FUNCTION "PALLET IMP.POST. SU USCI" : VOID
TITLE =
VERSION : 0.1
//KNOW_HOW_PROTECT

VAR_TEMP
  Error_block_move : INT ;
END_VAR
BEGIN
NETWORK
TITLE =

NETWORK
TITLE =Spostamento dati per pallet in transito tra ribaltat. e uscita
//- "Container Flag"
//- "Id TAG"
//- "FlagRibaltamento"
//- "Container_Id"
//- "Date LCB"
//- "Part Number"
//- "Quantity"
//- "Line Id"
//- "CIM"
//- "Colata Id"
//- "Material Of Test Flag"
//- "Lotto Id"
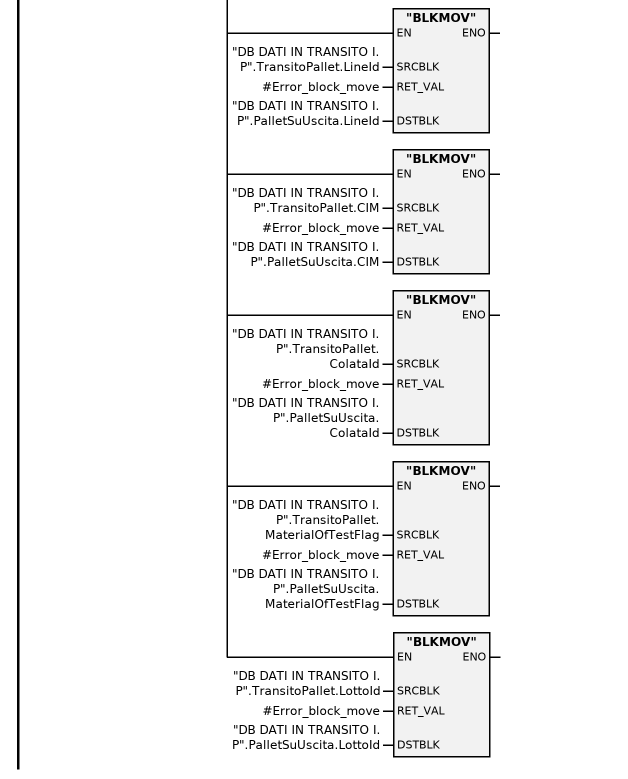
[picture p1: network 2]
      U     "M900.0";
      U     "DB SCAMBIO DATI PIANELLI".Pallet_I_P_su_uscita;
      =     L      2.0;
      U     L      2.0;
      SPBNB _001;
      CALL "BLKMOV" (
           SRCBLK                   := "DB DATI IN TRANSITO I. P".TransitoPallet.ContainerFlag,
           RET_VAL                  := #Error_block_move,
           DSTBLK                   := "DB DATI IN TRANSITO I. P".PalletSuUscita.ContainerFlag);
_001: NOP   0;
      U     L      2.0;
      SPBNB _002;
      CALL "BLKMOV" (
           SRCBLK                   := "DB DATI IN TRANSITO I. P".TransitoPallet.ID_TAG,
           RET_VAL                  := #Error_block_move,
           DSTBLK                   := "DB DATI IN TRANSITO I. P".PalletSuUscita.ID_TAG);
_002: NOP   0;
      U     L      2.0;
      SPBNB _003;
      CALL "BLKMOV" (
           SRCBLK                   := "DB DATI IN TRANSITO I. P".TransitoPallet.FlagRibaltamento,
           RET_VAL                  := #Error_block_move,
           DSTBLK                   := "DB DATI IN TRANSITO I. P".PalletSuUscita.FlagRibaltamento);
_003: NOP   0;
      U     L      2.0;
      SPBNB _004;
      CALL "BLKMOV" (
           SRCBLK                   := "DB DATI IN TRANSITO I. P".TransitoPallet.Container_Id,
           RET_VAL                  := #Error_block_move,
           DSTBLK                   := "DB DATI IN TRANSITO I. P".PalletSuUscita.Container_Id);
_004: NOP   0;
      U     L      2.0;
      SPBNB _005;
      CALL "BLKMOV" (
           SRCBLK                   := "DB DATI IN TRANSITO I. P".TransitoPallet.DateLCB,
           RET_VAL                  := #Error_block_move,
           DSTBLK                   := "DB DATI IN TRANSITO I. P".PalletSuUscita.DateLCB);
_005: NOP   0;
      U     L      2.0;
      SPBNB _006;
      CALL "BLKMOV" (
           SRCBLK                   := "DB DATI IN TRANSITO I. P".TransitoPallet.PartNumber,
           RET_VAL                  := #Error_block_move,
           DSTBLK                   := "DB DATI IN TRANSITO I. P".PalletSuUscita.PartNumber);
_006: NOP   0;
      U     L      2.0;
      SPBNB _007;
      CALL "BLKMOV" (
           SRCBLK                   := "DB DATI IN TRANSITO I. P".TransitoPallet.Quantity,
           RET_VAL                  := #Error_block_move,
           DSTBLK                   := "DB DATI IN TRANSITO I. P".PalletSuUscita.Quantity);
_007: NOP   0;
      U     L      2.0;
      SPBNB _008;
      CALL "BLKMOV" (
           SRCBLK                   := "DB DATI IN TRANSITO I. P".TransitoPallet.LineId,
           RET_VAL                  := #Error_block_move,
           DSTBLK                   := "DB DATI IN TRANSITO I. P".PalletSuUscita.LineId);
_008: NOP   0;
      U     L      2.0;
      SPBNB _009;
      CALL "BLKMOV" (
           SRCBLK                   := "DB DATI IN TRANSITO I. P".TransitoPallet.CIM,
           RET_VAL                  := #Error_block_move,
           DSTBLK                   := "DB DATI IN TRANSITO I. P".PalletSuUscita.CIM);
_009: NOP   0;
      U     L      2.0;
      SPBNB _00a;
      CALL "BLKMOV" (
           SRCBLK                   := "DB DATI IN TRANSITO I. P".TransitoPallet.ColataId,
           RET_VAL                  := #Error_block_move,
           DSTBLK                   := "DB DATI IN TRANSITO I. P".PalletSuUscita.ColataId);
_00a: NOP   0;
      U     L      2.0;
      SPBNB _00b;
      CALL "BLKMOV" (
           SRCBLK                   := "DB DATI IN TRANSITO I. P".TransitoPallet.MaterialOfTestFlag,
           RET_VAL                  := #Error_block_move,
           DSTBLK                   := "DB DATI IN TRANSITO I. P".PalletSuUscita.MaterialOfTestFlag);
_00b: NOP   0;
      U     L      2.0;
      SPBNB _00c;
      CALL "BLKMOV" (
           SRCBLK                   := "DB DATI IN TRANSITO I. P".TransitoPallet.LottoId,
           RET_VAL                  := #Error_block_move,
           DSTBLK                   := "DB DATI IN TRANSITO I. P".PalletSuUscita.LottoId);
_00c: NOP   0;
NETWORK
TITLE =Lettura Pallet su baia di scarico
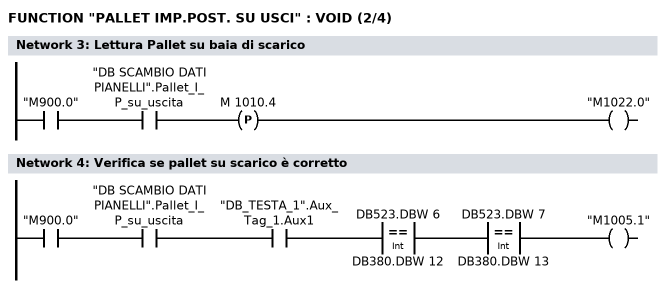
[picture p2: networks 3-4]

      U     "M900.0";
      U     "DB SCAMBIO DATI PIANELLI".Pallet_I_P_su_uscita;
      FP    M   1010.4;
      =     "M1022.0";
NETWORK
TITLE =Verifica se pallet su scarico è corretto

      U     "M900.0";
      U     "DB SCAMBIO DATI PIANELLI".Pallet_I_P_su_uscita;
      U     "DB_TESTA_1".Aux_Tag_1.Aux1;
      U(    ;
      L     DB523.DBW    6;
      L     DB380.DBW   12;
      ==I   ;
      )     ;
      U(    ;
      L     DB523.DBW    7;
      L     DB380.DBW   13;
      ==I   ;
      )     ;
      =     "M1005.1";
NETWORK
TITLE =Se pallet è corretto e ribaltato, aggiorno TAG
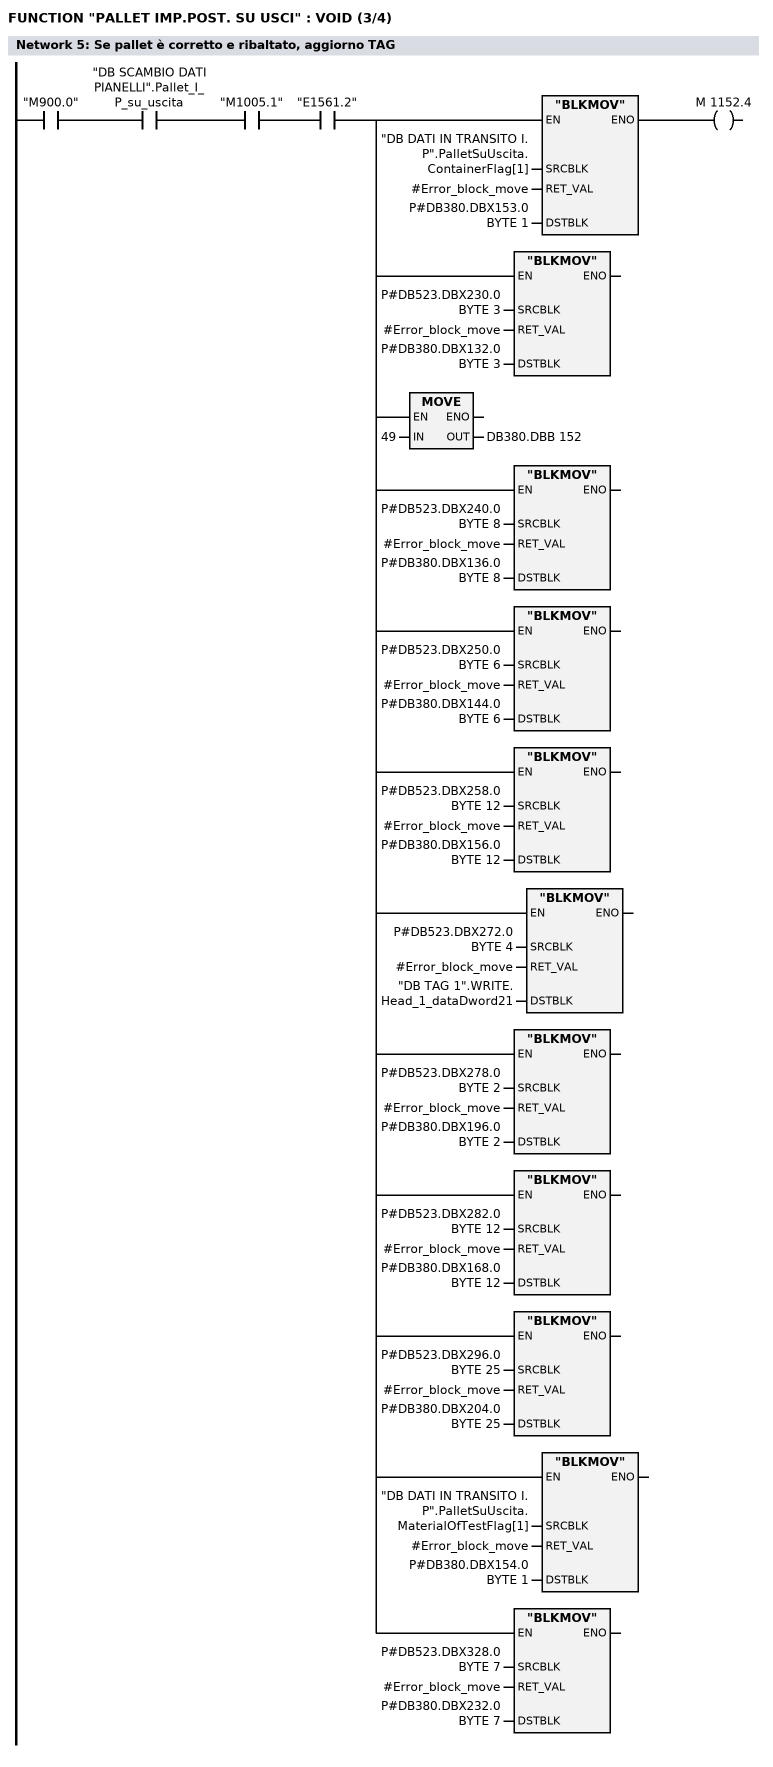
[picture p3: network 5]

      U     "M900.0";
      U     "DB SCAMBIO DATI PIANELLI".Pallet_I_P_su_uscita;
      U     "M1005.1";
      U     "E1561.2";
      =     L      2.0;
      U     L      2.0;
      SPBNB _00d;
      CALL "BLKMOV" (
           SRCBLK                   := "DB DATI IN TRANSITO I. P".PalletSuUscita.ContainerFlag[1],
           RET_VAL                  := #Error_block_move,
           DSTBLK                   := P#DB380.DBX153.0 BYTE 1);
_00d: U     BIE;
      =     M   1152.4;
      U     L      2.0;
      SPBNB _00e;
      CALL "BLKMOV" (
           SRCBLK                   := P#DB523.DBX230.0 BYTE 3,
           RET_VAL                  := #Error_block_move,
           DSTBLK                   := P#DB380.DBX132.0 BYTE 3);
_00e: NOP   0;
      U     L      2.0;
      SPBNB _00f;
      L     49;
      T     DB380.DBB  152;
_00f: NOP   0;
      U     L      2.0;
      SPBNB _010;
      CALL "BLKMOV" (
           SRCBLK                   := P#DB523.DBX240.0 BYTE 8,
           RET_VAL                  := #Error_block_move,
           DSTBLK                   := P#DB380.DBX136.0 BYTE 8);
_010: NOP   0;
      U     L      2.0;
      SPBNB _011;
      CALL "BLKMOV" (
           SRCBLK                   := P#DB523.DBX250.0 BYTE 6,
           RET_VAL                  := #Error_block_move,
           DSTBLK                   := P#DB380.DBX144.0 BYTE 6);
_011: NOP   0;
      U     L      2.0;
      SPBNB _012;
      CALL "BLKMOV" (
           SRCBLK                   := P#DB523.DBX258.0 BYTE 12,
           RET_VAL                  := #Error_block_move,
           DSTBLK                   := P#DB380.DBX156.0 BYTE 12);
_012: NOP   0;
      U     L      2.0;
      SPBNB _013;
      CALL "BLKMOV" (
           SRCBLK                   := P#DB523.DBX272.0 BYTE 4,
           RET_VAL                  := #Error_block_move,
           DSTBLK                   := "DB TAG 1".WRITE.Head_1_dataDword21);
_013: NOP   0;
      U     L      2.0;
      SPBNB _014;
      CALL "BLKMOV" (
           SRCBLK                   := P#DB523.DBX278.0 BYTE 2,
           RET_VAL                  := #Error_block_move,
           DSTBLK                   := P#DB380.DBX196.0 BYTE 2);
_014: NOP   0;
      U     L      2.0;
      SPBNB _015;
      CALL "BLKMOV" (
           SRCBLK                   := P#DB523.DBX282.0 BYTE 12,
           RET_VAL                  := #Error_block_move,
           DSTBLK                   := P#DB380.DBX168.0 BYTE 12);
_015: NOP   0;
      U     L      2.0;
      SPBNB _016;
      CALL "BLKMOV" (
           SRCBLK                   := P#DB523.DBX296.0 BYTE 25,
           RET_VAL                  := #Error_block_move,
           DSTBLK                   := P#DB380.DBX204.0 BYTE 25);
_016: NOP   0;
      U     L      2.0;
      SPBNB _017;
      CALL "BLKMOV" (
           SRCBLK                   := "DB DATI IN TRANSITO I. P".PalletSuUscita.MaterialOfTestFlag[1],
           RET_VAL                  := #Error_block_move,
           DSTBLK                   := P#DB380.DBX154.0 BYTE 1);
_017: NOP   0;
      U     L      2.0;
      SPBNB _018;
      CALL "BLKMOV" (
           SRCBLK                   := P#DB523.DBX328.0 BYTE 7,
           RET_VAL                  := #Error_block_move,
           DSTBLK                   := P#DB380.DBX232.0 BYTE 7);
_018: NOP   0;
NETWORK
TITLE =OK SCARICO PEDANA USCITA DA IMP_POSTERIORE
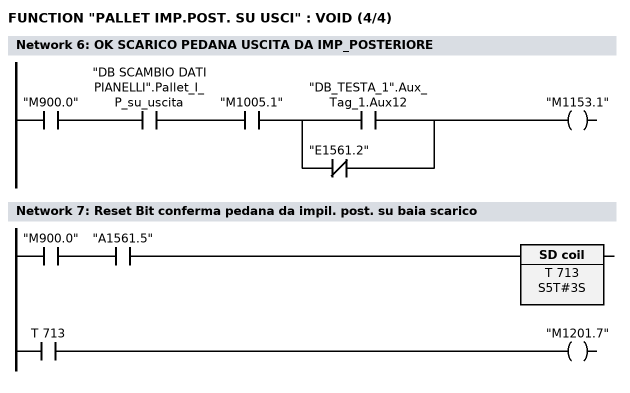
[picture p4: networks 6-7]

      U     "M900.0";
      U     "DB SCAMBIO DATI PIANELLI".Pallet_I_P_su_uscita;
      U     "M1005.1";
      U(    ;
      O     "DB_TESTA_1".Aux_Tag_1.Aux12;
      ON    "E1561.2";
      )     ;
      =     "M1153.1";
NETWORK
TITLE =Reset Bit conferma pedana da impil. post. su baia scarico

      U     "M900.0";
      U     "A1561.5";
      L     S5T#3S;
      SE    T    713;
      NOP   0;
      NOP   0;
      NOP   0;
      U     T    713;
      =     "M1201.7";
END_FUNCTION

